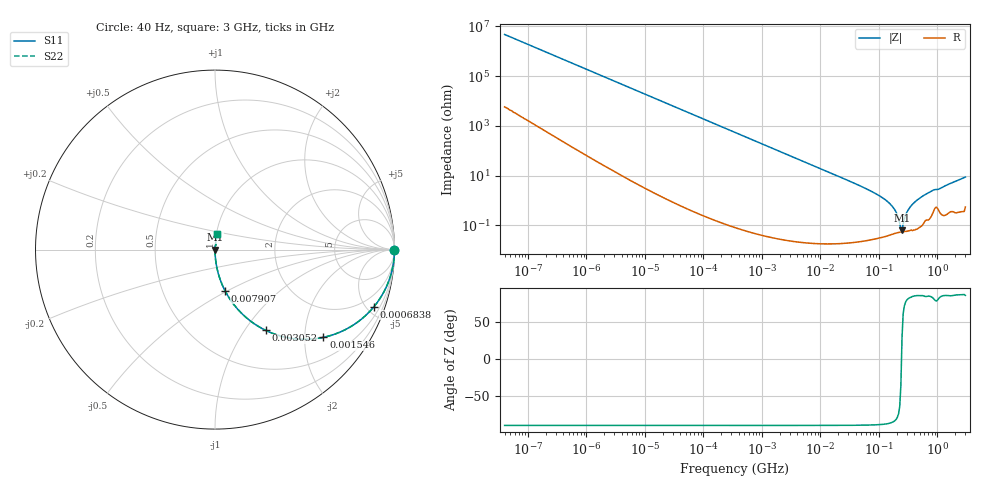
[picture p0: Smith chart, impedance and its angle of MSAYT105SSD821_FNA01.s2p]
! MSAYT105SSD821_FNA01  S-PARAMETER MODEL  ( General Type )
! Model Generated by TAIYO YUDEN Corporation (http://www.ty-top.com)
! Version 2.0
! TAIYO YUDEN Control No. 051115
! Copyright(c) 2005 TAIYO YUDEN CO.,LTD. All Rights Reserved.
! Product Description (link to TY-COMPAS)
! https://ds.yuden.co.jp/TYCOMPAS/or/detail?pn=MSAYT105SSD821KFNA01&u=M
! Products Name : Multilayer Ceramic Capacitors
! Characteristics :
!  Capacitance : 820 pF , Rated Voltage : 25V
!  Case Size : 1.0 x 0.5 / 0.039 x 0.02 [mm/inch] , Thickness : 0.5 / 0.02 [mm/inch]
!  (Conditions: Temperature = 25 degC , DC Bias Current/Voltage = 0A / 0V)
! External Node Assignments :
!  1  o---| |---o  2
! GND o---------o GND
! Frequency Range : 40Hz  -  3GHz  [ 401 STEP ]
# MHz S RI R 50
! Freq[MHz].  S11 Real  S11 Imag  S21 Real  S21 Imag  S12 Real  S12 Imag  S22 Real  S22 Imag
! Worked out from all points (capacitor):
!   401 points, 40 Hz to 3 GHz, reference 50 ohm
!   read as one part in series: C = 833 pF near 44 Hz
!   lowest |Z| = 62.3 mohm at 247.9 MHz (marker M1)
!   series resonance near 243 MHz, so ESL is about 510 pH
!   S11 on the Smith chart (normalised r, x): 40 Hz: open; 683.8 kHz: 1.00, -5.59; 1.546 MHz: 1.00, -2.47; 3.052 MHz: 1.00, -1.25; 7.907 MHz: 1.00, -0.48; 3 GHz: 1.01, +0.17
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4e-05  1 -2.09e-05  2.6e-08 2.09e-05  2.6e-08 2.09e-05  1 -2.09e-05
0.000187  1 -9.79e-05  7.4e-08 9.79e-05  7.4e-08 9.79e-05  1 -9.79e-05
0.000834  1 -0.000437  3.48e-07 0.000437  3.48e-07 0.000437  1 -0.000437
0.017386  0.9999 -0.0091  8.41e-05 0.0091  8.41e-05 0.0091  0.9999 -0.0091
0.111532  0.9966 -0.0582  0.0034 0.0582  0.0034 0.0582  0.9966 -0.0582
0.362475  0.9652 -0.1831  0.0348 0.1831  0.0348 0.1831  0.9652 -0.1831
0.683763  0.8864 -0.3172  0.1136 0.3172  0.1136 0.3172  0.8864 -0.3172
1.546262  0.6041 -0.4889  0.3959 0.4889  0.3959 0.4889  0.6041 -0.4889
3.052094  0.2815 -0.4496  0.7185 0.4496  0.7185 0.4496  0.2815 -0.4496
7.222098  0.0654 -0.247  0.9346 0.247  0.9346 0.247  0.0654 -0.247
7.907491  0.0552 -0.228  0.9448 0.228  0.9448 0.228  0.0552 -0.228
60.81113  0.0011 -0.0293  0.9989 0.0293  0.9989 0.0293  0.0011 -0.0293
104.7695  0.000529 -0.0147  0.9995 0.0147  0.9995 0.0147  0.000529 -0.0147
150.5692  0.000456 -0.00773  0.9995 0.00773  0.9995 0.00773  0.000456 -0.00773
188.875  0.000486 -0.00396  0.9995 0.00396  0.9995 0.00396  0.000486 -0.00396
226.4253  0.000528 -0.00109  0.9995 0.00109  0.9995 0.00109  0.000528 -0.00109
247.9136  0.000541 0.000308  0.9995 -0.000308  0.9995 -0.000308  0.000541 0.000308
259.4108  0.000554 0.00103  0.9994 -0.00103  0.9994 -0.00103  0.000554 0.00103
325.4065  0.000621 0.0046  0.9994 -0.0046  0.9994 -0.0046  0.000621 0.0046
467.657  0.00088 0.0111  0.9991 -0.0111  0.9991 -0.0111  0.00088 0.0111
805.711  0.00318 0.0241  0.9968 -0.0241  0.9968 -0.0241  0.00318 0.0241
3000  0.0128 0.0854  0.9872 -0.0854  0.9872 -0.0854  0.0128 0.0854
